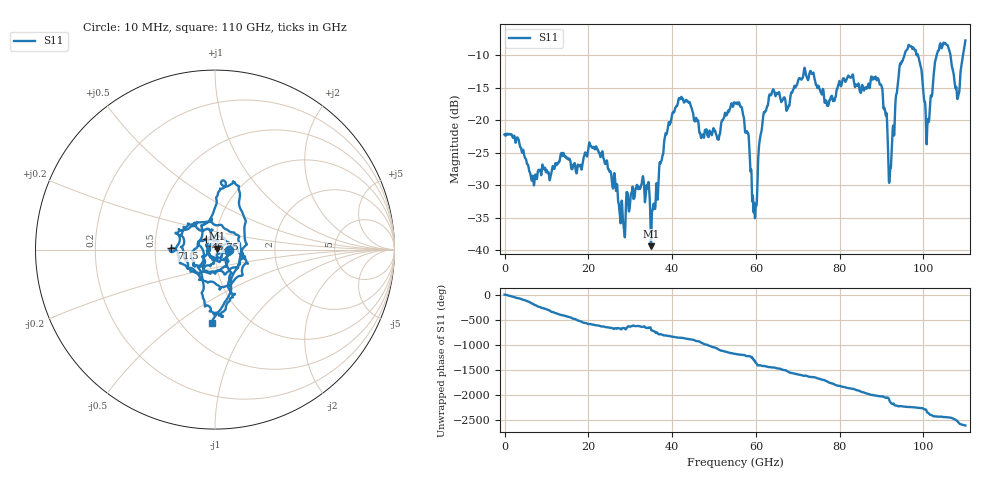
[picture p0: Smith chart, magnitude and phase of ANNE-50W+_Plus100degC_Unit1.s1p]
!Mini-Circuits Laboratory
!S-Parameters
!S1P File: Measurement
!Model: ANNE-50W+
!No.: Unit# 1 (U1_100°C)
!Run / Lot / Date Code: QN2409253 /  / 2409
!Fixture: N/A
!Network Analyzer: PNA-X N5242B;  Serial number: 74314
!Pin Outs: PORT<1> = pin<1>
!TEST CONDITIONS: Z:50 OHM SYSTEM, INPUT POWER = 0dBm, TEMP:25°C
!F-F adapter to 1FT F-M cable on Port 2 head. 1mm 1 PORT SmartCal
!Date: 9/5/2024 at 12:57:57 PM
# Hz  S  dB  R  50
!Frequency  S11 dB  S11 Deg
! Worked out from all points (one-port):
!   2208 points, 10 MHz to 110 GHz, reference 50 ohm
!   lowest |S11| = -39.3 dB at 34.95 GHz (marker M1), VSWR 1.02, Z = 51 + j0.519 ohm
!   |S11| at or under -10 dB: start of sweep to 95.46 GHz; 98.63 GHz to 103.2 GHz (4.52 GHz wide, 4.48 % of centre); 106.4 GHz to 109.4 GHz (3.001 GHz wide, 2.78 % of centre)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
!   S11 on the Smith chart (normalised r, x): 10 MHz: 1.17, +0.00; 46.75 GHz: 0.90, +0.11; 71.5 GHz: 0.61, +0.01; 110 GHz: 0.69, -0.68
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1e7  -22.24 0.2
6.7e9  -28.60 175.1
1.38e10  -25.52 -52.3
2.18e10  -24.09 107.1
2.755e10  -34.79 43.0
3.275e10  -29.67 75.2
3.495e10  -39.34 28.1
4.13e10  -17.57 -138.1
4.675e10  -22.14 130.4
5.505e10  -17.32 -103.5
5.795e10  -21.86 -150.0
5.965e10  -33.16 125.9
6.125e10  -21.91 23.3
6.305e10  -16.69 -9.1
6.88e10  -15.45 -131.1
7.15e10  -12.26 177.9
7.625e10  -16.34 96.7
7.965e10  -14.61 -20.1
8.255e10  -13.40 -75.1
8.96e10  -14.56 129.9
9.2e10  -28.07 20.6
9.425e10  -11.91 -69.5
9.63e10  -8.83 -85.0
9.9e10  -10.89 -102.5
1.01e11  -19.93 162.7
1.0445e11  -8.72 77.6
1.081e11  -16.75 -10.8
1.1e11  -7.77 -92.6
